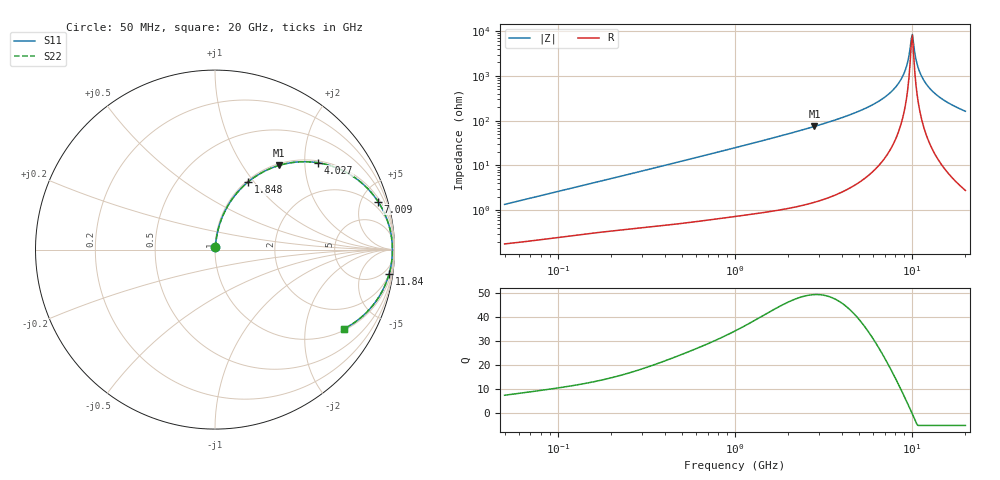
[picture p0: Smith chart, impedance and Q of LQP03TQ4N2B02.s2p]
!Murata Part Number: LQP03TQ4N2B02
!These Parameters are Measured in Series Mode Connection
!  o--[Z]--o
!Port1  Port2
!  o-------o
!Freq. Start=50[MHz] Stop=20[GHz], 401[Steps]
# Hz S RI R 50
!Freq.(Hz) S11(Real) S11(Imag) S21(Real) S21(Imag) S12(Real) S12(Imag) S22(Real) S22(Imag)
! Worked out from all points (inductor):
!   401 points, 50 MHz to 20 GHz, reference 50 ohm
!   read as one part in series: L = 4.22 nH near 51.52 MHz
!   highest Q = 49.4 at 2.811 GHz (marker M1), where L = 4.21 nH
!   self-resonance near 9.892 GHz
!   S11 on the Smith chart (normalised r, x): 50 MHz: 1.00, +0.03; 1.848 GHz: 1.02, +0.93; 4.027 GHz: 1.05, +2.34; 7.009 GHz: 1.29, +6.68; 11.84 GHz: 2, -14; 20 GHz: 1.06, -3.25
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5e7  0.00194 0.0133  0.9981 -0.0133  0.9981 -0.0133  0.00194 0.0133
1.364002e8  0.00408 0.0348  0.9959 -0.0348  0.9959 -0.0348  0.00408 0.0348
3.721004e8  0.0129 0.0914  0.9871 -0.0914  0.9871 -0.0914  0.0129 0.0914
1e9  0.0639 0.2305  0.9361 -0.2305  0.9361 -0.2305  0.0639 0.2305
1.848039e9  0.1844 0.3769  0.8156 -0.3769  0.8156 -0.3769  0.1844 0.3769
2.728004e9  0.343 0.4647  0.657 -0.4647  0.657 -0.4647  0.343 0.4647
2.810964e9  0.3585 0.4696  0.6415 -0.4696  0.6415 -0.4696  0.3585 0.4696
4.026975e9  0.5758 0.4834  0.4242 -0.4834  0.4242 -0.4834  0.5758 0.4834
5.515528e9  0.7812 0.3995  0.2188 -0.3995  0.2188 -0.3995  0.7812 0.3995
7.009217e9  0.9081 0.2679  0.0919 -0.2679  0.0919 -0.2679  0.9081 0.2679
7.442007e9  0.9321 0.2273  0.0679 -0.2273  0.0679 -0.2273  0.9321 0.2273
8.264682e9  0.9644 0.1507  0.0356 -0.1507  0.0356 -0.1507  0.9644 0.1507
8.907419e9  0.9794 0.0928  0.0206 -0.0928  0.0206 -0.0928  0.9794 0.0928
9.316812e9  0.9851 0.0572  0.0149 -0.0572  0.0149 -0.0572  0.9851 0.0572
9.745021e9  0.9881 0.0212  0.0119 -0.0212  0.0119 -0.0212  0.9881 0.0212
1.004137e10  0.9886 -0.00284  0.0114 0.00284  0.0114 0.00284  0.9886 -0.00284
1.019291e10  0.9884 -0.0149  0.0116 0.0149  0.0116 0.0149  0.9884 -0.0149
1.066139e10  0.9861 -0.0509  0.0139 0.0509  0.0139 0.0509  0.9861 -0.0509
1.098561e10  0.9831 -0.0748  0.0169 0.0748  0.0169 0.0748  0.9831 -0.0748
1.183995e10  0.9706 -0.1335  0.0294 0.1335  0.0294 0.1335  0.9706 -0.1335
1.460232e10  0.9001 -0.2834  0.0999 0.2834  0.0999 0.2834  0.9001 -0.2834
2e10  0.7214 -0.4399  0.2786 0.4399  0.2786 0.4399  0.7214 -0.4399
